FUNCTION FC 38 : VOID
TITLE =BLOCK CAM ELECTRONICS
AUTHOR : Esposito
FAMILY : EGAL_srl
NAME : C_ELECTR
VERSION : 0.1


VAR_TEMP
  CAMEN : BOOL ;
  CNTC0EN : BOOL ;
  CNTC1EN : BOOL ;
  CAMACT : BOOL ;
  RETVAL : INT ;
  DATAERR : BOOL ;
  JPCCEDG : BOOL ;
  INCCEDG : BOOL ;
END_VAR
BEGIN
NETWORK
TITLE =ENABLE CAMS
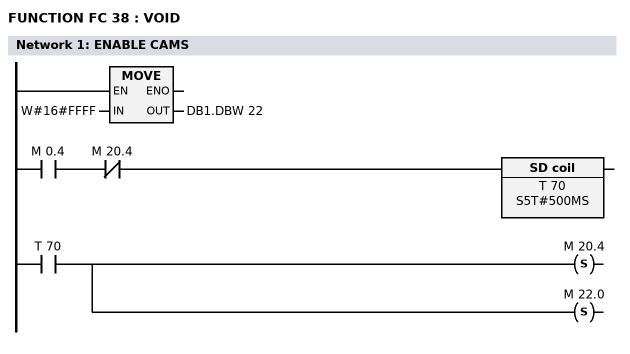
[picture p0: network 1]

      L     W#16#FFFF;
      T     DB1.DBW   22;
//;
      U     M      0.4;
      UN    M     20.4;
      L     S5T#500MS;
      SE    T     70;
      NOP   0;
      NOP   0;
      NOP   0;
      U     T     70;
      S     M     20.4;
      S     M     22.0;
NETWORK
TITLE =CAM ZERO - DIE AUTOMATION 38YV1

      UN    M     22.0;
      SPB   CAMZ;
//;
      L     W#16#0;
      T     DB1.DBW   86;
//;
      CALL FC   120 (
           WIN                      := DB15.DBW   22,
           WOUT                     := DB1.DBD   88);
//;
      CALL FC   120 (
           WIN                      := DB15.DBW   24,
           WOUT                     := DB1.DBD   92);
//;
      CALL FC    12 (
           DB_NO                    := DB     1,
           RET_VAL                  := #RETVAL,
           DATA_ERR                 := #DATAERR,
           JP_CCEDG                 := #JPCCEDG,
           IN_CCEDG                 := M     22.0);
//;
      UN    BIE;
      SPB   CAMZ;
//;
      S     M     22.1;
//;
CAMZ: U     M     22.1;
      L     S5T#1S;
      SE    T     71;
//;
      U     T     71;
      R     M     22.1;
      S     M     22.2;
NETWORK
TITLE =CAM ONE - DIE AUTOMATION 38YV2

      UN    M     22.2;
      SPB   CAMO;
//;
      L     W#16#1;
      T     DB1.DBW   86;
//;
      CALL FC   120 (
           WIN                      := DB15.DBW   26,
           WOUT                     := DB1.DBD   88);
//;
      CALL FC   120 (
           WIN                      := DB15.DBW   28,
           WOUT                     := DB1.DBD   92);
//;
      CALL FC    12 (
           DB_NO                    := DB     1,
           RET_VAL                  := #RETVAL,
           DATA_ERR                 := #DATAERR,
           JP_CCEDG                 := #JPCCEDG,
           IN_CCEDG                 := M     22.2);
//;
      UN    BIE;
      SPB   CAMO;
//;
      S     M     22.3;
//;
CAMO: U     M     22.3;
      L     S5T#1S;
      SE    T     72;
//;
      U     T     72;
      R     M     22.3;
      S     M     22.4;
NETWORK
TITLE =CAM TWO - DIE AUTOMATION 38YV3

      UN    M     22.4;
      SPB   CAMT;
//;
      L     W#16#2;
      T     DB1.DBW   86;
//;
      CALL FC   120 (
           WIN                      := DB15.DBW   30,
           WOUT                     := DB1.DBD   88);
//;
      CALL FC   120 (
           WIN                      := DB15.DBW   32,
           WOUT                     := DB1.DBD   92);
//;
      CALL FC    12 (
           DB_NO                    := DB     1,
           RET_VAL                  := #RETVAL,
           DATA_ERR                 := #DATAERR,
           JP_CCEDG                 := #JPCCEDG,
           IN_CCEDG                 := M     22.4);
//;
      UN    BIE;
      SPB   CAMT;
//;
      S     M     22.5;
//;
CAMT: U     M     22.5;
      L     S5T#1S;
      SE    T     73;
//;
      U     T     73;
      R     M     22.5;
      S     M     22.6;
NETWORK
TITLE =CAM THREE - DIE AUTOMATION 38YV4

      UN    M     22.6;
      SPB   CAMH;
//;
      L     W#16#3;
      T     DB1.DBW   86;
//;
      CALL FC   120 (
           WIN                      := DB15.DBW   34,
           WOUT                     := DB1.DBD   88);
//;
      CALL FC   120 (
           WIN                      := DB15.DBW   36,
           WOUT                     := DB1.DBD   92);
//;
      CALL FC    12 (
           DB_NO                    := DB     1,
           RET_VAL                  := #RETVAL,
           DATA_ERR                 := #DATAERR,
           JP_CCEDG                 := #JPCCEDG,
           IN_CCEDG                 := M     22.6);
//;
      UN    BIE;
      SPB   CAMH;
//;
      S     M     22.7;
//;
CAMH: U     M     22.7;
      L     S5T#1S;
      SE    T     74;
//;
      U     T     74;
      R     M     22.7;
      S     M     23.0;
NETWORK
TITLE =CAM FOUR - DIE AUTOMATION SPARE

      UN    M     23.0;
      SPB   CAMF;
//;
      L     W#16#4;
      T     DB1.DBW   86;
//;
      CALL FC   120 (
           WIN                      := DB15.DBW   38,
           WOUT                     := DB1.DBD   88);
//;
      CALL FC   120 (
           WIN                      := DB15.DBW   40,
           WOUT                     := DB1.DBD   92);
//;
      CALL FC    12 (
           DB_NO                    := DB     1,
           RET_VAL                  := #RETVAL,
           DATA_ERR                 := #DATAERR,
           JP_CCEDG                 := #JPCCEDG,
           IN_CCEDG                 := M     23.0);
//;
      UN    BIE;
      SPB   CAMF;
//;
      S     M     23.1;
//;
CAMF: U     M     23.1;
      L     S5T#1S;
      SE    T     75;
//;
      U     T     75;
      R     M     23.1;
      S     M     23.2;
NETWORK
TITLE =CAM FIVE - FEEDER START

      UN    M     23.2;
      SPB   CAMV;
//;
      L     W#16#5;
      T     DB1.DBW   86;
//;
      CALL FC   120 (
           WIN                      := DB15.DBW   42,
           WOUT                     := DB1.DBD   88);
//;
      CALL FC   120 (
           WIN                      := DB15.DBW   44,
           WOUT                     := DB1.DBD   92);
//;
      CALL FC    12 (
           DB_NO                    := DB     1,
           RET_VAL                  := #RETVAL,
           DATA_ERR                 := #DATAERR,
           JP_CCEDG                 := #JPCCEDG,
           IN_CCEDG                 := M     23.2);
//;
      UN    BIE;
      SPB   CAMV;
//;
      S     M     23.3;
//;
CAMV: U     M     23.3;
      L     S5T#1S;
      SE    T     76;
//;
      U     T     76;
      R     M     23.3;
      S     M     23.4;
NETWORK
TITLE =CAM SIX - STEP CONTROL

      UN    M     23.4;
      SPB   CAMX;
//;
      L     W#16#6;
      T     DB1.DBW   86;
//;
      CALL FC   120 (
           WIN                      := DB15.DBW   46,
           WOUT                     := DB1.DBD   88);
//;
      CALL FC   120 (
           WIN                      := DB15.DBW   48,
           WOUT                     := DB1.DBD   92);
//;
      CALL FC    12 (
           DB_NO                    := DB     1,
           RET_VAL                  := #RETVAL,
           DATA_ERR                 := #DATAERR,
           JP_CCEDG                 := #JPCCEDG,
           IN_CCEDG                 := M     23.4);
//;
      UN    BIE;
      SPB   CAMX;
//;
      S     M     23.5;
//;
CAMX: U     M     23.5;
      L     S5T#1S;
      SE    T     77;
//;
      U     T     77;
      R     M     23.5;
      S     M     23.6;
NETWORK
TITLE =CAM SEVEN - DIE SAFETY

      UN    M     23.6;
      SPB   CAMS;
//;
      L     W#16#7;
      T     DB1.DBW   86;
//;
      CALL FC   120 (
           WIN                      := DB15.DBW   50,
           WOUT                     := DB1.DBD   88);
//;
      CALL FC   120 (
           WIN                      := DB15.DBW   52,
           WOUT                     := DB1.DBD   92);
//;
      CALL FC    12 (
           DB_NO                    := DB     1,
           RET_VAL                  := #RETVAL,
           DATA_ERR                 := #DATAERR,
           JP_CCEDG                 := #JPCCEDG,
           IN_CCEDG                 := M     23.6);
//;
      UN    BIE;
      SPB   CAMS;
//;
      S     M     23.7;
//;
CAMS: U     M     23.7;
      L     S5T#1S;
      SE    T     78;
//;
      U     T     78;
      R     M     23.7;
      S     M     24.0;
NETWORK
TITLE =CAM EIGHT - UDP STOP

      UN    M     24.0;
      SPB   CAMG;
//;
      L     W#16#8;
      T     DB1.DBW   86;
//;
      CALL FC   120 (
           WIN                      := DB15.DBW   54,
           WOUT                     := DB1.DBD   88);
//;
      CALL FC   120 (
           WIN                      := DB15.DBW   56,
           WOUT                     := DB1.DBD   92);
//;
      CALL FC    12 (
           DB_NO                    := DB     1,
           RET_VAL                  := #RETVAL,
           DATA_ERR                 := #DATAERR,
           JP_CCEDG                 := #JPCCEDG,
           IN_CCEDG                 := M     24.0);
//;
      UN    BIE;
      SPB   CAMG;
//;
      S     M     24.1;
//;
CAMG: U     M     24.1;
      L     S5T#1S;
      SE    T     79;
//;
      U     T     79;
      R     M     24.1;
      S     M     24.2;
NETWORK
TITLE =CAM NINE - ROBOT 1 START

      UN    M     24.2;
      SPB   CAMN;
//;
      L     W#16#9;
      T     DB1.DBW   86;
//;
      CALL FC   120 (
           WIN                      := DB15.DBW   58,
           WOUT                     := DB1.DBD   88);
//;
      CALL FC   120 (
           WIN                      := DB15.DBW   60,
           WOUT                     := DB1.DBD   92);
//;
      CALL FC    12 (
           DB_NO                    := DB     1,
           RET_VAL                  := #RETVAL,
           DATA_ERR                 := #DATAERR,
           JP_CCEDG                 := #JPCCEDG,
           IN_CCEDG                 := M     24.2);
//;
      UN    BIE;
      SPB   CAMN;
//;
      S     M     24.3;
//;
CAMN: U     M     24.3;
      L     S5T#1S;
      SE    T     80;
//;
      U     T     80;
      R     M     24.3;
      S     M     24.4;
NETWORK
TITLE =CAM TEN - ROBOT 2 START

      UN    M     24.4;
      SPB   CAME;
//;
      L     W#16#A;
      T     DB1.DBW   86;
//;
      CALL FC   120 (
           WIN                      := DB15.DBW   62,
           WOUT                     := DB1.DBD   88);
//;
      CALL FC   120 (
           WIN                      := DB15.DBW   64,
           WOUT                     := DB1.DBD   92);
//;
      CALL FC    12 (
           DB_NO                    := DB     1,
           RET_VAL                  := #RETVAL,
           DATA_ERR                 := #DATAERR,
           JP_CCEDG                 := #JPCCEDG,
           IN_CCEDG                 := M     24.4);
//;
      UN    BIE;
      SPB   CAME;
//;
      S     M     24.5;
//;
CAME: U     M     24.5;
      L     S5T#1S;
      SE    T     81;
//;
      U     T     81;
      R     M     24.5;
      S     M     24.6;
NETWORK
TITLE =CAM ELEVEN - ROBOT 1 SAFETY

      UN    M     24.6;
      SPB   CAML;
//;
      L     W#16#B;
      T     DB1.DBW   86;
//;
      CALL FC   120 (
           WIN                      := DB15.DBW   66,
           WOUT                     := DB1.DBD   88);
//;
      CALL FC   120 (
           WIN                      := DB15.DBW   68,
           WOUT                     := DB1.DBD   92);
//;
      CALL FC    12 (
           DB_NO                    := DB     1,
           RET_VAL                  := #RETVAL,
           DATA_ERR                 := #DATAERR,
           JP_CCEDG                 := #JPCCEDG,
           IN_CCEDG                 := M     24.6);
//;
      UN    BIE;
      SPB   CAML;
//;
      S     M     24.7;
//;
CAML: U     M     24.7;
      L     S5T#1S;
      SE    T     82;
//;
      U     T     82;
      R     M     24.7;
      S     M     25.0;
NETWORK
TITLE =CAM TWELVE - ROBOT 2 SAFETY

      UN    M     25.0;
      SPB   CAMW;
//;
      L     W#16#C;
      T     DB1.DBW   86;
//;
      CALL FC   120 (
           WIN                      := DB15.DBW   70,
           WOUT                     := DB1.DBD   88);
//;
      CALL FC   120 (
           WIN                      := DB15.DBW   72,
           WOUT                     := DB1.DBD   92);
//;
      CALL FC    12 (
           DB_NO                    := DB     1,
           RET_VAL                  := #RETVAL,
           DATA_ERR                 := #DATAERR,
           JP_CCEDG                 := #JPCCEDG,
           IN_CCEDG                 := M     25.0);
//;
      UN    BIE;
      SPB   CAMW;
//;
      S     M     25.1;
//;
CAMW: U     M     25.1;
      L     S5T#1S;
      SE    T     83;
//;
      U     T     83;
      R     M     25.1;
      S     M     25.2;
NETWORK
TITLE =CAM THIRTEEN - CAM PROGRESSIVE DIE

      UN    M     25.2;
      SPB   CAMR;
//;
      L     W#16#D;
      T     DB1.DBW   86;
//;
      CALL FC   120 (
           WIN                      := DB15.DBW   74,
           WOUT                     := DB1.DBD   88);
//;
      CALL FC   120 (
           WIN                      := DB15.DBW   76,
           WOUT                     := DB1.DBD   92);
//;
      CALL FC    12 (
           DB_NO                    := DB     1,
           RET_VAL                  := #RETVAL,
           DATA_ERR                 := #DATAERR,
           JP_CCEDG                 := #JPCCEDG,
           IN_CCEDG                 := M     25.2);
//;
      UN    BIE;
      SPB   CAMR;
//;
      S     M     25.3;
//;
CAMR: U     M     25.3;
      L     S5T#1S;
      SE    T     84;
//;
      U     T     84;
      R     M     25.3;
      S     M     25.4;
NETWORK
TITLE =SET BLOCK DATA CAM

      SET   ;
      =     #CAMEN;
      CLR   ;
      =     #CNTC0EN;
      CLR   ;
      =     #CNTC1EN;
//;
      UN    M     25.4;
      SPB   _001;
//;
      CALL FC     0 (
           DB_NO                    := DB     1,
           CAM_EN                   := #CAMEN,
           CNTC0_EN                 := #CNTC0EN,
           CNTC1_EN                 := #CNTC1EN,
           CAM_ACT                  := #CAMACT);
//;
      U     BIE;
      S     M     25.5;
//;
_001: NOP   0;
NETWORK
TITLE =RESET BLOCK DATA CAMS
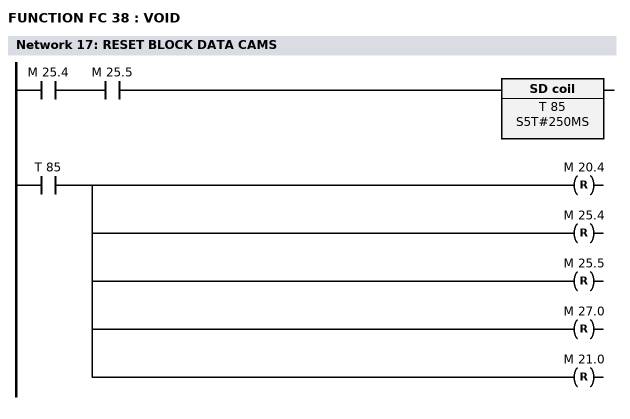
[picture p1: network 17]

      U     M     25.4;
      U     M     25.5;
      L     S5T#250MS;
      SE    T     85;
      NOP   0;
      NOP   0;
      NOP   0;
      U     T     85;
      R     M     20.4;
      R     M     25.4;
      R     M     25.5;
      R     M     27.0;
      R     M     21.0;
END_FUNCTION

